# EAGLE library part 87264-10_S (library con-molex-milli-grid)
RECEPTACAL
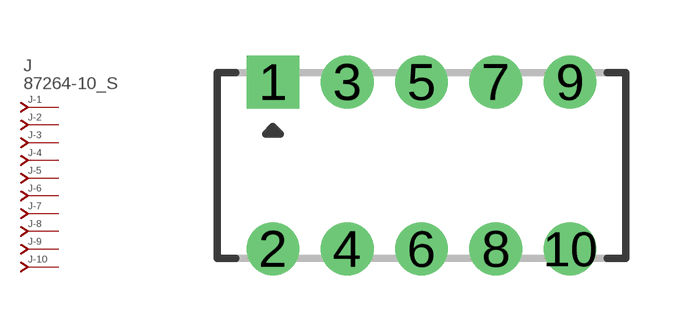
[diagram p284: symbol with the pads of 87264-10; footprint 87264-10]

Designator prefix J; gates -1=J-NV -2=J-N -3=J-N -4=J-N -5=J-N -6=J-N -7=J-N -8=J-N -9=J-N -10=J-N

## 87264-10_S  [87264-10]
1  -1:J  pas
2  -2:J  pas
3  -3:J  pas
4  -4:J  pas
5  -5:J  pas
6  -6:J  pas
7  -7:J  pas
8  -8:J  pas
9  -9:J  pas
10  -10:J  pas

## Footprint 87264-10 (pad centres in mm)
RECEPTACAL Dual Row, Side Entry
drill 0.914 square: 1 -4,2.25
drill 0.914: 2 -4,-2.25; 3 -2,2.25; 4 -2,-2.25; 5 0,2.25; 6 0,-2.25; 7 2,2.25; 8 2,-2.25; 9 4,2.25; 10 4,-2.25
